PROGRAM MAIN
VAR
	// crossing with 4 traffic lights
	fbCrossing 		: FB_Crossing;
	// single traffic light
	fbTrafficLight 	: FB_SingleTrafficLight := (sInName := 'Traffic Light Single');
END_VAR

fbCrossing.M_Cycle();

fbTrafficLight.M_Cycle();

END_PROGRAM
